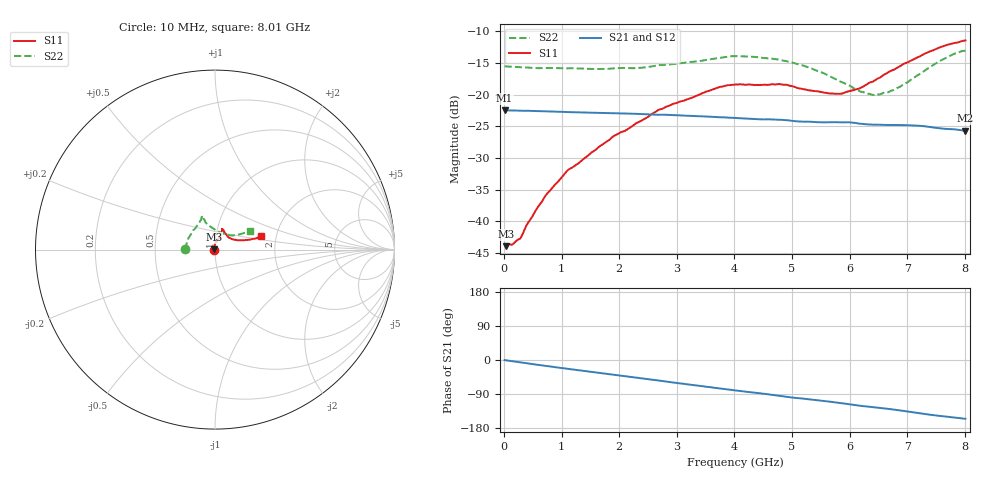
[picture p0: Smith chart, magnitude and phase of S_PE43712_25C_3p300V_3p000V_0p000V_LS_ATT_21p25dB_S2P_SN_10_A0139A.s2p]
! DEVICE ID: PE43712
! File Path: z:\PE43713\PE43713_CHAR_NOM_04292014\AMB\3p300\LS_ATT_21p25dB\PE43713_AMB_3p300V_3p000V_0p000V_LS_ATT_21p25dB_S2P_SN_10_A0139A.s2p
! Serial: 10
! Lot: A0139A
! Temp: 25C
! VDD: 3.300
! VSS: 0.000
! Control_Hi: 3.000
! Control_Lo: 0.000
! Attenuation Step: 21.25dB
! Port 1: RF1
! Port 2: RF2
! ThroughPath:1-2
! IDD: 0.0001470907
! ISS: -8.97e-008
#  Hz  S  RI  R  50
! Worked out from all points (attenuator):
!   801 points, 10 MHz to 8.01 GHz, reference 50 ohm
!   highest |S21| = -22.49 dB at 10 MHz (marker M1); lowest = -25.7 dB at 8.01 GHz (marker M2)
!   lowest |S11| = -43.9 dB at 30 MHz (marker M3), VSWR 1.01, Z = 49.4 + j0.136 ohm
!   |S11| at or under -10 dB: start of sweep to end of sweep
!   |S22| runs from -20.1 to -13.1 dB; largest |S21 - S12| = 0.00028
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1e7  -0.00661 0.000553  0.0751 -0.000401  0.0751 -0.000375  -0.1671 0.00117
3e7  -0.00623 0.00138  0.075 -0.000938  0.0751 -0.000954  -0.1666 0.00277
1.5e8  -0.0054 0.00377  0.0747 -0.00442  0.0747 -0.00442  -0.165 0.0103
2.8e8  -0.00459 0.00571  0.0742 -0.00805  0.0742 -0.0081  -0.1632 0.0167
4.2e8  -0.00437 0.00878  0.0735 -0.0119  0.0734 -0.012  -0.1613 0.0238
7.4e8  -0.00401 0.0159  0.0708 -0.0201  0.0708 -0.0202  -0.1564 0.0416
1.1e9  -0.00254 0.0251  0.0669 -0.0286  0.0669 -0.0286  -0.1492 0.06
1.35e9  -9.19e-05 0.0303  0.0638 -0.034  0.0638 -0.034  -0.1434 0.071
1.91e9  0.00867 0.0464  0.0553 -0.0448  0.0553 -0.0448  -0.1259 0.1003
2.68e9  0.0268 0.0706  0.0406 -0.0561  0.0406 -0.0561  -0.0964 0.1403
3.71e9  0.039 0.1064  0.0179 -0.0638  0.0178 -0.0638  -0.0745 0.1785
4.01e9  0.0402 0.1128  0.0112 -0.0644  0.0112 -0.0644  -0.0748 0.1863
4.79e9  0.0439 0.1125  -0.0051 -0.063  -0.00515 -0.063  -0.0648 0.176
5.35e9  0.0565 0.0909  -0.0155 -0.0589  -0.0155 -0.0588  -0.052 0.151
5.87e9  0.0771 0.0665  -0.0247 -0.055  -0.0246 -0.055  -0.0187 0.1235
6.17e9  0.0954 0.0578  -0.0302 -0.0506  -0.03 -0.0507  0.00811 0.1062
6.38e9  0.1125 0.0554  -0.0323 -0.048  -0.0322 -0.048  0.0304 0.0952
6.68e9  0.1414 0.0519  -0.0363 -0.0446  -0.0362 -0.0446  0.0646 0.0826
7e9  0.1707 0.0534  -0.041 -0.04  -0.0409 -0.0399  0.0964 0.0787
7.55e9  0.2253 0.0624  -0.0456 -0.0293  -0.0456 -0.0293  0.1573 0.0911
7.81e9  0.2443 0.0699  -0.0468 -0.0252  -0.0468 -0.0252  0.1825 0.1012
8.01e9  0.2556 0.0761  -0.0469 -0.0219  -0.0468 -0.0219  0.1943 0.1059
